PROGRAM MAIN
VAR
	nCount1 : INT;
	nCount2 : INT;
END_VAR

nCount1 := nCount1 + 1;

nCount2 := nCount2 + 5;

IF nCount1 = 500 THEN
	nCount1 := 0;
END_IF

IF nCount2 = 4000 THEN
	nCount2 := 0;
END_IF

END_PROGRAM
